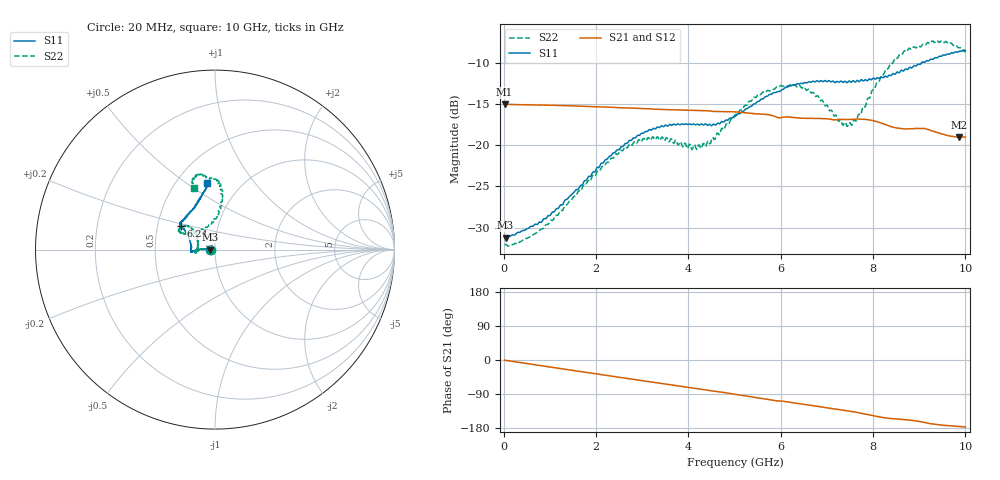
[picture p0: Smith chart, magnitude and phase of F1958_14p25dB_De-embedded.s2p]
! Integrated Device Technology
! Corporate Headquarters
! 6024 Silver Creek Valley Road
! San Jose, CA 95138  USA
! Phone:  1-408-284-8200
! Toll Free:  1-800-223-1366
! Webpage:  http://www.idt.com/
! Timing and RF Division
! 515 Groton Road, Suite 102
! Westford, MA 01886-6024
! Device:  F1958
! Description: 7-bit 0.25 dB Digital Step Attenuator
! Frequency:  0.001 -  6.000 GHz
! Package:  4x4 mm Thin QFN Plastic Package: 24 pin
! Ports:  2 RF, 12 DC
!  Pin  1  = D0
!  Pin  2  = VDD
!  Pin  3  = VMODE
!  Pin  4  = GND
!  Pin  5  = RF1  =  Port 1
!  Pin  6  = GND
!  Pin  7  = GND
!  Pin  8  = GND
!  Pin  9  = GND
!  Pin 10  = GND
!  Pin 11  = GND
!  Pin 12  = GND
!  Pin 13  = GND
!  Pin 14  = RF2  =  Port 2
!  Pin 15  = GND
!  Pin 16  = LE
!  Pin 17  = CLK
!  Pin 18  = DATA
!  Pin 19  = D6
!  Pin 20  = D5
!  Pin 21  = D4
!  Pin 22  = D3
!  Pin 23  = D2
!  Pin 24  = D1
! State:  57
! Atten State:  14.25 dB
! Voltage:  +3.30 Volts
! Current:  0.258 mA
! Data:  The device was measured on a F1958 evaluation board which has
!  individual transmission lines to the RF pins.  Data was collected
!  using a calibrated network analyzer.  The evaluation board was
!  de-embedded using Automatic Fixture Removal (AFR).
!  The reference plane is the edge of the package pin.
! Misc:
!  Action Tracker AT0419
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# GHz S dB R 50
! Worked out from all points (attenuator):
!   500 points, 20 MHz to 10 GHz, reference 50 ohm
!   highest |S21| = -15.05 dB at 20 MHz (marker M1); lowest = -19.0 dB at 9.86 GHz (marker M2)
!   lowest |S11| = -31.2 dB at 40 MHz (marker M3), VSWR 1.06, Z = 47.3 - j0.0744 ohm
!   |S11| at or under -10 dB: start of sweep to 9.057 GHz
!   |S22| runs from -32.2 to -7.3 dB; largest |S21 - S12| = 0.00046
!   S11 on the Smith chart (normalised r, x): 20 MHz: 0.95, -0.00; 6.24 GHz: 0.66, +0.18; 10 GHz: 0.70, +0.61
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0.02  -31.21 -178.3  -15.05 -0.5  -15.05 -0.5  -32.09 -178.4
0.04  -31.22 -178.4  -15.06 -0.9  -15.06 -0.9  -32.03 -177.8
0.32  -30.57 177.6  -15.10 -6.1  -15.10 -6.0  -31.90 177.7
0.84  -29.18 176.0  -15.15 -15.6  -15.15 -15.6  -30.15 178.3
1.7  -24.82 177.3  -15.30 -31.1  -15.29 -31.1  -25.17 177.5
2.6  -20.07 -179.0  -15.49 -47.3  -15.47 -47.3  -20.47 -177.6
2.92  -18.82 -176.3  -15.55 -53.0  -15.54 -53.1  -19.37 -174.3
3.36  -17.86 -174.2  -15.67 -60.9  -15.67 -61.0  -19.28 -170.3
4.24  -17.59 -179.7  -15.81 -76.4  -15.82 -76.5  -20.01 167.6
4.5  -17.66 174.4  -15.91 -81.4  -15.92 -81.4  -19.41 152.2
5.02  -16.51 159.9  -15.98 -90.6  -15.99 -90.6  -16.28 138.8
5.54  -14.66 149.6  -16.22 -100.2  -16.24 -100.2  -13.86 140.0
6.24  -12.77 145.5  -16.63 -112.5  -16.65 -112.5  -12.87 151.2
6.68  -12.31 143.3  -16.77 -120.1  -16.78 -120.0  -13.65 152.9
7.3  -12.23 137.0  -16.89 -131.4  -16.90 -131.3  -16.95 131.5
7.5  -12.28 134.2  -16.90 -135.2  -16.90 -135.1  -17.27 113.4
7.68  -12.25 131.1  -16.85 -139.0  -16.84 -139.0  -16.30 96.9
8.34  -11.55 115.3  -17.68 -153.8  -17.68 -153.9  -10.61 81.9
8.68  -10.90 108.6  -18.03 -157.3  -18.04 -157.3  -8.57 86.4
9.26  -9.58 100.8  -18.25 -168.3  -18.25 -168.3  -7.50 99.2
9.86  -8.65 96.4  -19.04 -175.3  -19.07 -175.2  -8.22 108.3
10  -8.54 96.5  -19.00 -177.0  -19.02 -176.9  -8.74 109.1
